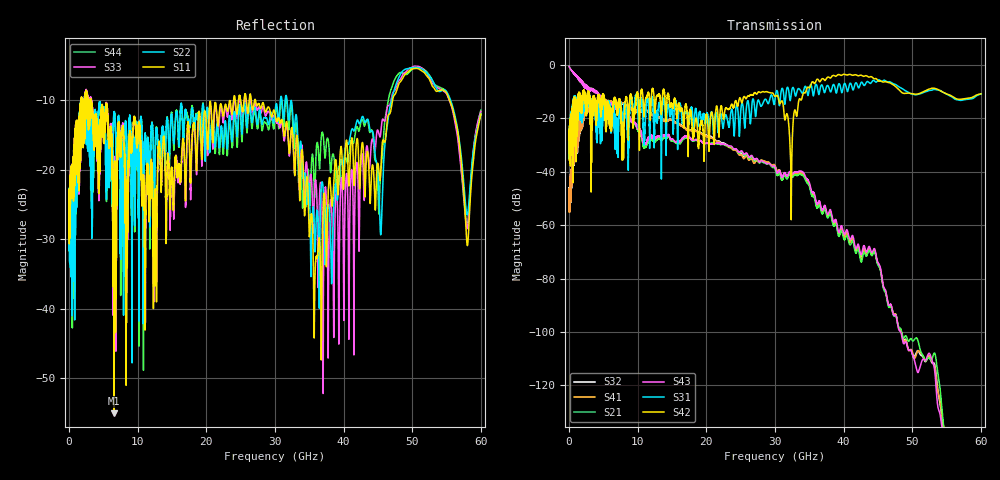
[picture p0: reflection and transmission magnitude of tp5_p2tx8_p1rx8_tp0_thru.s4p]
! 100G CR Analysis
! File: tp5_p2tx8_p1rx8_tp0_thru
! Description: 2m Cu Cable, OSFP, TP0-TP5
! Port Mapping
! Port1 -- P1RX8N
! Port2 -- P2TX8N
! Port3 -- P1RX8P
! Port4 -- P2TX8P
# GHz S MA R 50.00
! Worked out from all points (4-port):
!   6000 points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, 10 MHz to 60 GHz, reference 50 ohm
!   strongest paths, dB at 10 MHz, 15.01 GHz, 30.01 GHz, 45.01 GHz, 60 GHz:
!     S42: -28.1, -15.5, -11.8, -5.9, -10.8
!     S31: -27.9, -18.4, -12.9, -5.7, -10.8
!     S43: -0.5, -27.9, -38.2, -74.1, -171.7
!     S21: -0.5, -28.3, -38.9, -75.1, -183.8
!     S41: -46.6, -20.7, -37.7, -74.5, -177.9
!     S32: -46.4, -20.6, -37.8, -74.7, -176.2
!   lowest |S11| = -55.1 dB at 6.54 GHz (marker M1), VSWR 1.00, Z = 49.8 - j0.0264 ohm
!   |S11| at or under -10 dB: 3.194 GHz to 23.96 GHz (20.77 GHz wide, 153 % of centre); 27.16 GHz to 47.14 GHz (19.98 GHz wide, 53.8 % of centre); 55.42 GHz to end of sweep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
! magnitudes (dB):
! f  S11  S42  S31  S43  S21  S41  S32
! 10 MHz  -23.9  -28.1  -27.9  -0.5  -0.5  -46.6  -46.4
! 2.28 GHz  -9.6  -10.3  -11.8  -8.5  -8.4  -15.4  -15.5
! 6.54 GHz  -55.1  -14.2  -15.8  -15.2  -15.2  -14.7  -14.8
! 29.44 GHz  -12.2  -10.5  -11.3  -37.6  -37.9  -37.4  -37.6
! 32.32 GHz  -14.7  -40.3  -11.9  -40.4  -41.4  -40.7  -40.9
! 36.17 GHz  -32.6  -5.3  -8.3  -52.0  -53.5  -52.7  -52.8
! 60 GHz  -12.0  -10.8  -10.8  -171.7  -183.8  -177.9  -176.2
